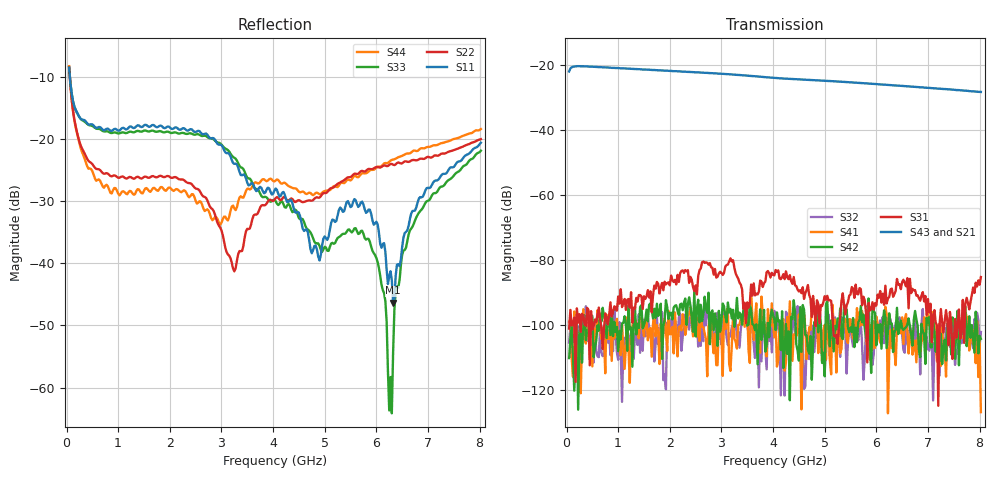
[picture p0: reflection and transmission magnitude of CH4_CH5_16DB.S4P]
!Agilent Technologies,E5071C,MY46316741,A.11.02
!Date: Mon Jun 01 11:47:15 2026
!Data & Calibration Information:
!1:CH4 INPUT 2:CH4 OUTPUT 3:CH5 INPUT 4:CH5 OUTPUT
!Freq	S11:SOLT4(ON)	S12:SOLT4(ON)	S13:SOLT4(ON)	S14:SOLT4(ON)
!	S21:SOLT4(ON)	S22:SOLT4(ON)	S23:SOLT4(ON)	S24:SOLT4(ON)
!	S31:SOLT4(ON)	S32:SOLT4(ON)	S33:SOLT4(ON)	S34:SOLT4(ON)
!	S41:SOLT4(ON)	S42:SOLT4(ON)	S43:SOLT4(ON)	S44:SOLT4(ON)
!PortZ  Port1:50+j0  Port2:50+j0  Port3:50+j0  Port4:50+j0
!Above PortZ is port z conversion or system Z0 setting when saving the data.
!When reading, reference impedance value at option line is always used.
# Hz S dB R 50
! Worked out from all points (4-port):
!   320 points, 50 MHz to 8.025 GHz, reference 50 ohm
!   strongest paths, dB at 50 MHz, 2.05 GHz, 4.05 GHz, 6.05 GHz, 8.025 GHz:
!     S43: -21.9, -21.7, -23.9, -25.8, -28.2
!     S21: -21.9, -21.8, -24.0, -26.0, -28.3
!     S31: -101.2, -86.2, -83.1, -91.6, -85.3
!     S42: -110.3, -98.4, -101.7, -102.3, -104.3
!     S41: -99.1, -100.7, -99.4, -103.9, -126.9
!     S32: -105.5, -98.6, -101.4, -101.3, -102.2
!   lowest |S11| = -46.3 dB at 6.325 GHz (marker M1), VSWR 1.01, Z = 49.7 - j0.396 ohm
!   |S11| at or under -10 dB: 64.76 MHz to end of sweep
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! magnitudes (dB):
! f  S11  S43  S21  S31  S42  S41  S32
! 50 MHz  -8.5  -21.9  -21.9  -101.2  -110.3  -99.1  -105.5
! 725 MHz  -18.6  -20.6  -20.7  -101.3  -97.4  -102.9  -108.9
! 3.25 GHz  -24.0  -22.9  -23.0  -82.3  -100.6  -104.2  -96.7
! 5.725 GHz  -30.1  -25.5  -25.7  -94.0  -99.3  -95.8  -106.4
! 6.325 GHz  -46.3  -26.1  -26.4  -91.4  -108.4  -101.3  -100.8
! 6.65 GHz  -32.9  -26.5  -26.7  -85.8  -100.4  -103.7  -100.0
! 8.025 GHz  -20.6  -28.2  -28.3  -85.3  -104.3  -126.9  -102.2
